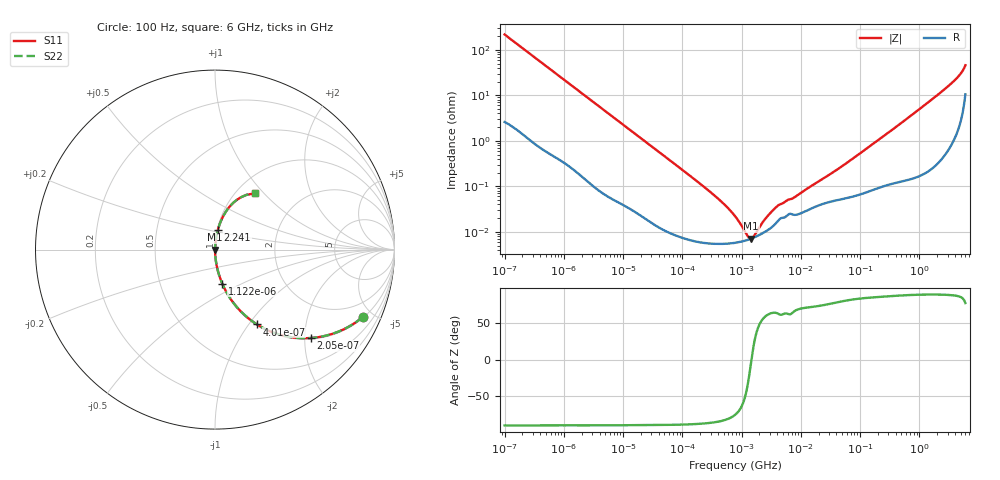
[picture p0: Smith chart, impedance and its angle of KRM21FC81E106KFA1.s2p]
!Murata Part Number: KRM21FC81E106KFA1
!These Parameters are Measured in Series Mode Connection
!Data Generated on Jan 08, 2026
!  o--ll--o
!Port1  Port2
!  o------o
!Operation Temp=25[degC], DC Bias Voltage=0[V]
!Freq. Start=100[Hz] Stop=6[GHz] 401[Steps]
# Hz S RI R 50
!Freq.(Hz) S11(Real) S11(Imag) S21(Real) S21(Imag) S12(Real) S12(Imag) S22(Real) S22(Imag)
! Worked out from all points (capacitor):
!   401 points, 100 Hz to 6 GHz, reference 50 ohm
!   read as one part in series: C = 7.3 uF near 109 Hz
!   lowest |Z| = 7.1 mohm at 1.45 MHz (marker M1)
!   series resonance near 1.469 MHz, so ESL is about 1.6 nH
!   S11 on the Smith chart (normalised r, x): 100 Hz: 1.05, -4.34; 205 Hz: 1.03, -2.14; 401 Hz: 1.01, -1.10; 1.122 kHz: 1.01, -0.40; 2.241 GHz: 1.01, +0.23; 6 GHz: 1.21, +0.89
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100  0.8222 -0.3765  0.1778 0.3765  0.1778 0.3765  0.8222 -0.3765
205  0.5327 -0.4926  0.4673 0.4926  0.4673 0.4926  0.5327 -0.4926
401  0.2343 -0.4172  0.7657 0.4172  0.7657 0.4172  0.2343 -0.4172
627  0.1135 -0.3104  0.8865 0.3104  0.8865 0.3104  0.1135 -0.3104
1122  0.0403 -0.1892  0.9597 0.1892  0.9597 0.1892  0.0403 -0.1892
2008  0.0138 -0.1095  0.9862 0.1095  0.9862 0.1095  0.0138 -0.1095
6433  0.00175 -0.0349  0.9982 0.0349  0.9982 0.0349  0.00175 -0.0349
40335  0.000157 -0.00569  0.9998 0.00569  0.9998 0.00569  0.000157 -0.00569
330837  5.52e-05 -0.000666  0.9999 0.000666  0.9999 0.000666  5.52e-05 -0.000666
774597  5.74e-05 -0.000214  0.9999 0.000214  0.9999 0.000214  5.74e-05 -0.000214
1159002  6.43e-05 -7.4e-05  0.9999 7.4e-05  0.9999 7.4e-05  6.43e-05 -7.4e-05
1449809  7.09e-05 -4e-06  0.9999 4e-06  0.9999 4e-06  7.09e-05 -4e-06
1813585  8.04e-05 6.4e-05  0.9999 -6.4e-05  0.9999 -6.4e-05  8.04e-05 6.4e-05
2713602  0.000107 0.00019  0.9999 -0.00019  0.9999 -0.00019  0.000107 0.00019
4060267  0.000172 0.000331  0.9998 -0.000331  0.9998 -0.000331  0.000172 0.000331
7599586  0.000237 0.000508  0.9998 -0.000508  0.9998 -0.000508  0.000237 0.000508
1.555665e7  0.000333 0.000994  0.9997 -0.000994  0.9997 -0.000994  0.000333 0.000994
4.983056e7  0.000532 0.00272  0.9995 -0.00272  0.9995 -0.00272  0.000532 0.00272
3.124326e8  0.00134 0.0157  0.9987 -0.0157  0.9987 -0.0157  0.00134 0.0157
2.240541e9  0.016 0.1105  0.984 -0.1105  0.984 -0.1105  0.016 0.1105
4.385646e9  0.0693 0.224  0.9307 -0.224  0.9307 -0.224  0.0693 0.224
6e9  0.2216 0.3134  0.7784 -0.3134  0.7784 -0.3134  0.2216 0.3134
